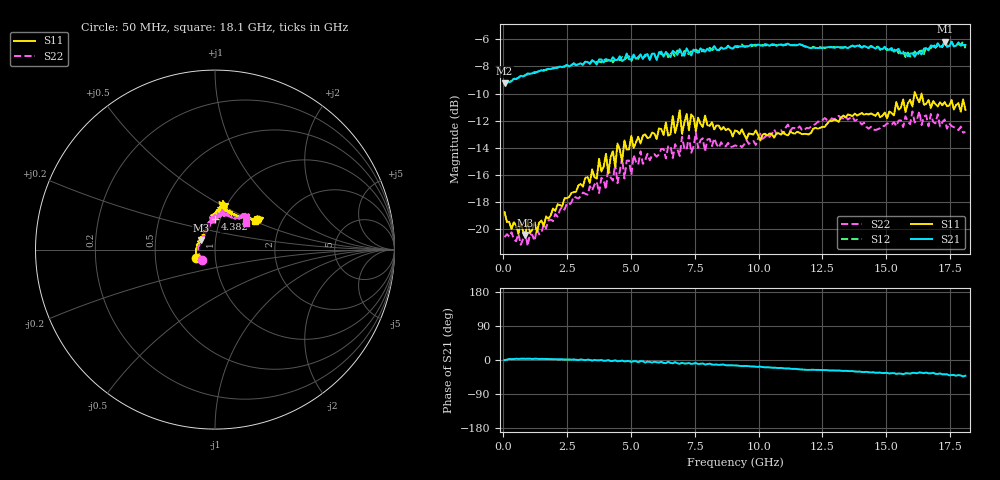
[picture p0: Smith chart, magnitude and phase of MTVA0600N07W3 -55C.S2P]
! Network Analyzer HP8720D.06.14 Serial No. US36140669
!  8 Jul 2005  12:26:31
! Frequency  S11  S21  S12  S22
# HZ  S  DB R 50
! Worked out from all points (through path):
!   201 points, 50 MHz to 18.1 GHz, reference 50 ohm
!   highest |S21| = -6.17 dB at 17.29 GHz (marker M1); lowest = -9.3 dB at 50 MHz (marker M2)
!   group delay of S21, straight-line fit = 7.51 ps
!   lowest |S11| = -20.5 dB at 862.2 MHz (marker M3), VSWR 1.21, Z = 42.5 + j4.61 ohm
!   |S11| at or under -10 dB: start of sweep to 16.11 GHz; 16.14 GHz to end of sweep
!   |S22| runs from -21.3 to -11.3 dB; largest |S21 - S12| = 0.026
!   S11 on the Smith chart (normalised r, x): 50 MHz: 0.81, -0.08; 4.382 GHz: 0.94, +0.33; 18.1 GHz: 1.47, +0.51
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5e7  -18.77 -156.5  -9.25 -0.4  -9.24 -0.1  -20.62 -142.5
8.6225e8  -20.46 145.5  -8.66 3.0  -8.62 3.2  -20.25 150.8
3.1185e9  -16.89 102.3  -7.85 0.7  -7.87 0.3  -17.33 107.5
4.021e9  -14.47 94.2  -7.45 -1.9  -7.61 -0.5  -17.09 98.5
4.11125e9  -15.91 93.5  -7.53 -0.2  -7.56 -2.3  -15.41 97.0
4.29175e9  -14.26 96.5  -7.31 -2.6  -7.70 -2.1  -16.44 91.3
4.382e9  -15.44 90.3  -7.52 -0.8  -7.47 -2.8  -15.17 97.3
4.47225e9  -13.70 84.8  -7.52 -3.3  -7.38 -1.2  -16.64 100.8
4.65275e9  -15.05 85.0  -7.60 -1.6  -7.30 -3.1  -14.76 99.0
4.743e9  -13.46 87.2  -7.48 -3.6  -7.48 -2.0  -16.29 95.3
5.104e9  -14.02 89.0  -7.12 -2.9  -7.23 -4.5  -14.54 90.0
6.09675e9  -12.58 80.9  -6.99 -6.9  -6.94 -6.5  -14.50 86.2
6.7285e9  -12.91 84.9  -6.97 -5.6  -7.28 -6.9  -13.75 79.6
6.909e9  -11.23 80.8  -6.72 -9.8  -6.94 -7.6  -14.61 78.1
6.99925e9  -12.99 81.0  -7.09 -7.3  -7.21 -9.8  -13.20 78.7
7.17975e9  -11.51 84.7  -6.66 -9.2  -7.05 -7.9  -14.18 73.5
7.54075e9  -12.78 75.5  -6.91 -8.0  -6.74 -11.0  -12.90 80.1
9.075e9  -12.73 73.1  -6.53 -14.4  -6.51 -14.4  -13.83 65.6
1.21435e10  -12.60 51.3  -6.59 -25.8  -6.54 -25.8  -12.34 52.5
1.512175e10  -11.34 32.7  -6.77 -35.5  -6.55 -35.2  -12.28 48.0
1.728775e10  -10.64 37.0  -6.17 -37.7  -6.08 -38.0  -11.92 48.0
1.81e10  -11.20 35.7  -6.41 -41.4  -6.65 -41.8  -12.85 40.4
